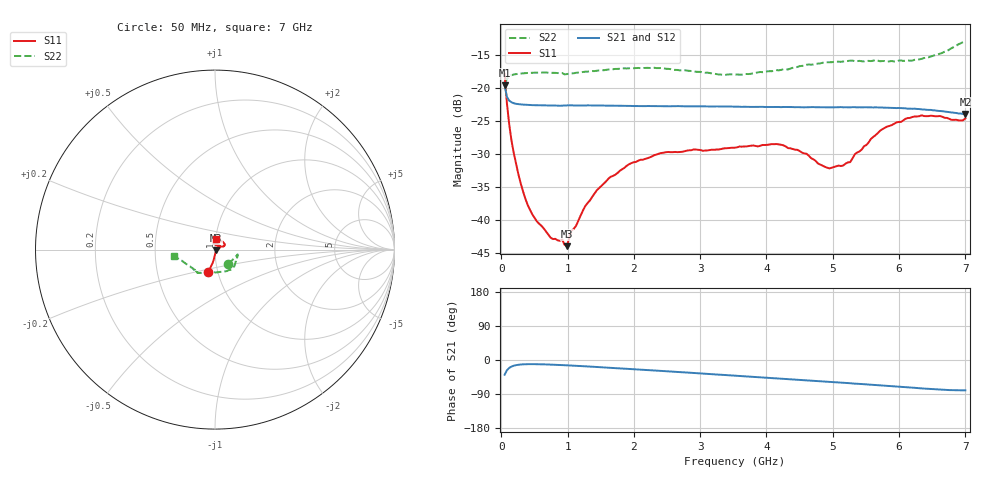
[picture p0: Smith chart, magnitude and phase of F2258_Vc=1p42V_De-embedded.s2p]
! Integrated Device Technology
! Corporate Headquarters
! 6024 Silver Creek Valley Road
! San Jose, CA 95138  USA
! Phone:  1-408-284-8200
! Toll Free:  1-800-223-1366
! Webpage:  http://www.idt.com/
! Timing and RF Division
! 515 Groton Road, Suite 102
! Westford, MA 01886-6024
! Device:  F2258
! Description: Voltage Variable RF Attenuator
! Frequency:  50.0 -  6000.00 MHz
! Package:  3x3 mm Thin QFN Plastic Package: 16 pin
! Ports:  2 RF, 2 DC
!  Pin  1  = NC
!  Pin  2  = NC
!  Pin  3  = RF2  = Port 2
!  Pin  4  = GND
!  Pin  5  = Vdd
!  Pin  6  = NC
!  Pin  7  = VCTRL
!  Pin  8  = NC
!  Pin  9  = GND
!  Pin 10  = RF1  = Port 1
!  Pin 11  = NC
!  Pin 12  = NC
!  Pin 13  = NC
!  Pin 14  = NC
!  Pin 15  = NC
!  Pin 16  = NC
! Vcntrl:  1.420 Volts
! Vdd:  +3.300 Volts
! Current:  1.162 mA
! Data:  The device was measured on a the F2258 evaluation board which has
!  individual transmission lines to the RF pins.  Data was collected
!  using a calibrated network analyzer.  The evaluation board was
!  de-embedded using a TRL calibration technique.
!  The reference plane is the edge of the package pin.
! Misc:  SN 10
!  Action Tracker AT0285
! Date Measured:  2014-12-10
! Date:  2016-01-13  MJV
! Note:
!  Integrated Device Technology supplies this data as a sample of measured
!  data at the package pin for this product.  Your particular data for this
!  product may vary.
!  Data was taken at 25 degrees C.
!  Integrated Device Technology reserves the right to change this data at anytime.
!Freq_(GHz)  S11M_(dB)  S11P_(deg)  S21M_(dB)  S21P_(deg)  S12M_(dB)  S12P_(deg)  S22M_(dB)  S22P_(deg)
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# GHz S dB R 50
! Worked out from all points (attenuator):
!   201 points, 50 MHz to 7 GHz, reference 50 ohm
!   highest |S21| = -19.56 dB at 50 MHz (marker M1); lowest = -23.9 dB at 7 GHz (marker M2)
!   lowest |S11| = -43.9 dB at 988.2 MHz (marker M3), VSWR 1.01, Z = 50.6 - j0.309 ohm
!   |S11| at or under -10 dB: start of sweep to end of sweep
!   |S22| runs from -19.3 to -12.7 dB; largest |S21 - S12| = 0.00071
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0.05  -17.80 -106.5  -19.56 -38.8  -19.51 -38.7  -19.29 -46.9
0.08475  -22.28 -100.3  -21.29 -27.1  -21.23 -27.0  -18.57 -24.1
0.15425  -27.95 -94.5  -22.11 -17.3  -22.08 -17.2  -18.00 -14.8
0.2585  -33.06 -87.6  -22.40 -12.6  -22.36 -12.6  -17.79 -12.1
0.36275  -36.73 -79.8  -22.49 -11.2  -22.45 -11.2  -17.70 -12.7
0.467  -39.10 -68.0  -22.55 -10.9  -22.51 -10.9  -17.64 -13.8
0.745  -42.65 -38.9  -22.62 -12.1  -22.56 -12.1  -17.66 -19.1
0.91875  -42.92 -10.0  -22.63 -13.5  -22.58 -13.5  -17.68 -23.4
0.98825  -43.93 -28.7  -22.59 -14.0  -22.60 -14.0  -17.85 -24.6
1.05775  -41.59 -15.9  -22.58 -14.6  -22.59 -14.6  -17.74 -25.9
1.2315  -38.53 -1.2  -22.61 -16.2  -22.59 -16.3  -17.53 -29.5
1.6485  -33.42 10.4  -22.63 -20.7  -22.63 -20.7  -17.14 -37.4
1.96125  -31.34 20.0  -22.67 -24.0  -22.67 -24.0  -16.94 -43.1
2.37825  -29.90 31.3  -22.71 -28.4  -22.72 -28.4  -16.92 -51.3
3.525  -29.00 83.0  -22.78 -41.3  -22.76 -41.4  -17.92 -87.2
4.18525  -28.49 102.1  -22.83 -48.8  -22.80 -48.9  -17.27 -110.7
4.7065  -30.76 91.5  -22.84 -54.8  -22.82 -54.9  -16.38 -121.5
4.94975  -32.14 71.6  -22.89 -57.6  -22.85 -57.7  -16.05 -124.1
5.15825  -31.69 50.7  -22.88 -60.2  -22.85 -60.3  -15.93 -126.1
5.85325  -25.71 21.5  -22.96 -68.7  -22.95 -68.7  -15.91 -133.2
6.33975  -24.09 28.9  -23.19 -75.0  -23.18 -75.0  -15.53 -145.5
7  -24.56 83.7  -23.90 -80.0  -23.90 -80.1  -12.74 -171.6
